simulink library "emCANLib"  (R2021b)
settings: Solver=VariableStepAuto  StartTime=0.0  StopTime=10.0  RelTol=1e-3
undefined symbols (not defined in the file or in its folder): Big, bool, Endian, Little, Seq2

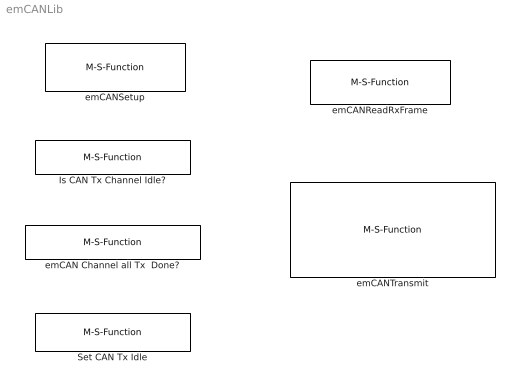
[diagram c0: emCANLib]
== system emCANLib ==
  Is CAN Tx Channel Idle? : M-S-Function  Tag=isCANTx_Idle  FunctionName=isCANTx_Idle2  Parameters=c_CAN_DeviceNo, c_ChannelName,c_sampleTime  mask(Is CAN bus Transmission Channel in "Idle" State){c_CAN_DeviceNo=1, c_ChannelName=Channel B, c_sampleTime=-1}
      mask prompts: c_CAN_DeviceNo "Peripheral CAN bus  Number:"; c_ChannelName "Transmit Channel:"; c_sampleTime "Sample time in sec (-1 for inherited):"
      mask help: Judge whether embedded CAN Bus transmission Channel is in "Idle" State. CAN bus peripheral has 3 Channels ( Channel A, B, C ) for transmitting. Every channels has as many as 31 Sequences (Seq0 to Seq30). Seq0 has higher priority than Seq30. Sequences run step by step from Seq0 to Seq30. 3 Channels can transmit at the same time. Usually we assign different channel into different sample time. So we can transmit 3 groups of CAN Packets in different periods. We do any "CAN BusTransmit " in One Channel must be under condition : Transmission Channel is in "Idle" State. This block is for this purpose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
      mask init:
      | try
      |     set_param(gcs,'Lock',"off");
      |     set_param(gcbh,'MaskSelfModifiable',"on");
      | end
  Set CAN Tx Idle : M-S-Function  Tag=setCANTx2Idle  FunctionName=setCANTx2Idle2  Parameters=c_CAN_DeviceNo, c_ChannelName  mask(set CAN bus Tx Channel into "Idle" State){c_CAN_DeviceNo=1, c_ChannelName=Channel A}
      mask prompts: c_CAN_DeviceNo "Peripheral CAN bus  Number:"; c_ChannelName "Transmit Channel:"
      mask help: set embedded CAN Bus Tx one Channel into "Idle" State. CAN bus peripheral has 3 Channels ( Channel A, B, C ) for transmitting. Every channels has as many as 31 Sequences (Seq0 to Seq30). Seq0 has higher priority than Seq30. Sequences run step by step from Seq0 to Seq30. 3 Channels can be transmitted at the same time. Usually we assign different channel into different sample time. So we can transmit 3 groups of CAN Packets in different periods. We do any "CAN BusTransmit " in One Channel must be under condition : Transmit Channel is in "Idle" State. However, when you call any "Transmit" block b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
      mask init:
      | try
      |     set_param(gcs,'Lock',"off");
      |     set_param(gcbh,'MaskSelfModifiable',"on");
      | end
  emCAN Channel all Tx  Done? : M-S-Function  FunctionName=emCANChannelAllTxDone2  Parameters=c_CAN_DeviceNo, c_ChannelName,c_sampleTime  mask(emCAN bus Channel  all transmissions done?){c_CAN_DeviceNo=1, c_ChannelName=Channel A, c_sampleTime=-1}
      mask prompts: c_CAN_DeviceNo "Peripheral CAN bus  Number:"; c_ChannelName "Transmit Channel:"; c_sampleTime "Sample time in sec (-1 for inherited):"
      mask help: Judge whether all transmission Sequences are done for embedded CAN Bus one Channel. Its output connects input port "En" of block "setCANTx2Idle".
      mask init:
      | try
      | set_param(gcs,'Lock',"off");
      | set_param(gcbh,'MaskSelfModifiable',"on");
      | end
  emCANReadRxFrame : M-S-Function  FunctionName=emCANReadRxFrame2  Parameters=c_CAN_DeviceNo,c_SettingFormat,c_ReceivedType , c_CANID, c_RTR, c_DataType,c_Endian,c_OutputQty,c_OutputType,c_sampleTime  mask(emCANReadRxFrame){c_CAN_DeviceNo=1, c_SettingFormat=CAN ID  in Decimal Data format, c_ReceivedType=Standard 11 bits CAN ID short frame, c_CANID=4, c_RTR=off, c_DataType=[int8*3 bool*4  bool uint32 ], c_Endian=Little-Endian, c_OutputQty=[3  4  1  1], c_OutputType=[2  8  8  7], c_sampleTime=-1}
      mask prompts: c_CAN_DeviceNo "Peripheral CAN bus  Number:"; c_SettingFormat "Settings CAN ID format"; c_ReceivedType "Received CAN Packet type"; c_CANID "CAN ID for received frame(s)"; c_RTR "Remote Frame"; c_DataType "Data type"; c_Endian "Endian"; c_OutputQty "OutputQty"; c_OutputType "OutputDataType"; c_sampleTime "Sample time in sec (-1 for inherited):"
      mask help: Read CAN bus received Data or Remote frame. For data frame, it will keep previous reading data if CAN bus controller didn't receive Data packets. For remote frame, it will output "true" if CAN bus controller receives remote frame. And after this time's reading, it will output "false" if CAN bus controller won't receive remote frame in next sample time.
      mask init:
      | try
      | set_param(gcs,'Lock',"off");
      | set_param(gcbh,'MaskSelfModifiable',"on");
      | end
  emCANSetup : M-S-Function  Tag=emCANBus  FunctionName=emCANSetup2  Parameters=c_CAN_DeviceNo,c_saved_SettingFormat,c_SettingFormat,c_Mask0,c_Mask1,c_Mask2,c_CANID_short,c_CANID_long,c_FrameNoWay,c_MaxFrameQty,c_enableSync,c_Sync_RxCANID,c_Com_Fault_detection_Time,c_ASeq_QTY,c_BSeq_QTY,c_CSeq_QTY,c_RxStdShort_listData,c_RxExtShort_listData,c_RxStdLong_listData,c_RxExtLong_listData,c_RxStdSyncData,c_RxExtSyncData,c_txChaanelA_DataLength,c_txChaanelB_DataLength,c_txChaanelC_Da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  mask(emCAN Setup){c_CAN_DeviceNo=1, c_saved_SettingFormat=1, c_SettingFormat=Settings in Hex Data format, c_Mask0=5X, c_Mask1=82, c_Mask2=129X, c_CANID_short=[4,6,7,5X,6X], c_CANID_long=[6E,502X], c_FrameNoWay=1-based frame No, c_MaxFrameQty=8, c_enableSync=on, c_Sync_RxCANID=43, c_Com_Fault_detection_Time=88, c_ASeq_QTY=31, c_BSeq_QTY=0, c_CSeq_QTY=0, c_RxStdShort_listData=4, c_RxExtShort_listData=5, c_RxStdLong_listData=110, c_RxExtLong_listData=-1, c_RxStdSyncData=67, c_RxExtSyncData=-1, c_txChaanelA_DataLength="", c_txChaanelB_DataLength="", c_txChaanelC_DataLength="", c_sampleTime=-1}
      mask prompts: c_CAN_DeviceNo "Peripheral CAN bus  Number:"; c_saved_SettingFormat "setting old format"; c_SettingFormat "Settings input data format"; c_Mask0 "Mask0:"; c_Mask1 "Mask1:"; c_Mask2 "Mask2:"; c_CANID_short "Rx CAN ID for short frame or RTR"; c_CANID_long "Rx CAN ID for long frame"; c_FrameNoWay "Frame Number"; c_MaxFrameQty "Max frame Qty for long frame Rx/Tx"; c_enableSync "Sync Enable"; c_Sync_RxCANID "Sync Rx CAN ID"; c_Com_Fault_detection_Time "CAN bus communication fault detection time in ms:"; c_ASeq_QTY "Max Sequence Qty for CAN BUS transmit A Channel"; c_BSeq_QTY "Max Sequence Qty for CAN BUS transmit B Channel"; c_CSeq_QTY "Max Sequence Qty for CAN BUS transmit C Channel"; c_RxStdShort_listData "RxStdCANIDShort Data Value"; c_RxExtShort_listData "RxExtCANIDShort Data Value"; c_RxStdLong_listData "RxStdCANIDLong Data Value"; c_RxExtLong_listData "RxExtCANIDLong Data Value"; c_RxStdSyncData "RxSyncStdCANIDData Value -1 = Disable"; c_RxExtSyncData "RxSyncExtCANIDData Value , -1 =disable"; c_txChaanelA_DataLength "TxMaxDLC_Vector4ChannelA"; c_txChaanelB_DataLength "TxMaxDLC_Vector4ChannelB"; c_txChaanelC_DataLength "TxMaxDLC_Vector4ChannelC"; c_sampleTime "Sample time in sec (-1 for inherited):"
      mask help: Set up peripheral CAN bus controller. ALL CAN ID settings can be in Hex or Decimal. CAN Bus Transmission uses Channel conception. There are 3 Transmission Channels: Channel A, Channel B and Channel C. Every Channel can have as many as 31 sequences (Seq No is from 0 to 30). Small Sequence No has higher priority for transmit. Every Sequence transmits one CAN bus RTR/Data frame. Or every Sequence can also transmit multiple frames with the same CAN ID but different frame No in 1st data. In one channel, transmit CAN bus frame one by one according to Sequence No from 0 to 30. All Channels can run at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
      mask init:
      | try
      | set_param(gcs,'Lock',"off");
      | set_param(gcbh,'MaskSelfModifiable',"on");
      | end
  emCANTransmit : M-S-Function  Tag=emCANBUSTx  FunctionName=emCANTransmit2  Parameters=c_CAN_DeviceNo,c_SettingFormat,c_TxChannel,c_SeqNo,c_TransmittedType,c_CANID,c_RTR,c_DataType,c_Endian,c_NeedResponse,c_Timeout,c_ResponseCANIDType,c_CANID_Response,c_ResposeDataType,c_InputDataQty,c_InputType,c_OutputDataQty,c_OutputType,c_currentHex  mask(emCANTransmit){c_CAN_DeviceNo=1, c_SettingFormat=CAN ID  in Decimal Data format, c_TxChannel=Channel A, c_SeqNo=Seq2, c_TransmittedType=Standard 11 bits CAN ID long frame, c_CANID=103, c_RTR=off, c_DataType=[int8*3 bool*6 int8*8  ], c_Endian=Big-Endian, c_NeedResponse=on, c_Timeout=50, c_ResponseCANIDType=Standard 11 bits CAN ID short frame, c_CANID_Response=4, c_ResposeDataType=[int8*2  bool bool*6 uint16*2 ], c_InputDataQty=[3  6  8], c_InputType=[2  8  2], c_OutputDataQty=[2  1  6  2], c_OutputType=[2  8  8  5], c_currentHex=off}
      mask prompts: c_CAN_DeviceNo "Peripheral CAN bus  Number:"; c_SettingFormat "Settings CAN ID format"; c_TxChannel "Transmit Channel No:"; c_SeqNo "Transmit Sequence No:"; c_TransmittedType "Transmitted CAN Packet type"; c_CANID "CAN ID for transmitted frame(s)"; c_RTR "Transmit Remote Frame"; c_DataType "Transmitted data type"; c_Endian "Endian"; c_NeedResponse "Need response to this transmitted sequence"; c_Timeout "Time out for response in ms"; c_ResponseCANIDType "Response CAN Packet Type"; c_CANID_Response "CAN ID for response frame(s)"; c_ResposeDataType "Response data type"; c_InputDataQty "InputQty"; c_InputType "InputDataType"; c_OutputDataQty "OutputDataQty"; c_OutputType "OutputDataType"; c_currentHex "Current we use Hex for CAN ID"
      mask help: Transmit CAN bus Data or Remote frame by one sequence from Channel A or Channel B or Channel C. We can transmit CAN Bus Data/Remote frame in 3 different Channels at the same time. (Of cause, you'd better configure 3 buffers for transmitting in GUI software like Microchip MCC and STM32CubeIDE). In general, you can set 3 Channels into different sample time. Inside every channels, transmitting is in serial by Sequences. Every channel has maximum 31 Sequences: Seq0 to Seq30. Seq0 is the most highest priority, Seq30 is the most lowest priority. Before you transmitting any frame, you must make sure 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
      mask init:
      | try
      | set_param(gcs,'Lock',"off");
      | set_param(gcbh,'MaskSelfModifiable',"on");
      | end
